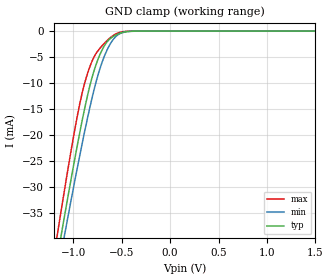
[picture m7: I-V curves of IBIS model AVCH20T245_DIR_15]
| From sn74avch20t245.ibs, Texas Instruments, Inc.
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[Model]   AVCH20T245_DIR_15
Model_type  Input
Vinl=0.49
Vinh=1.04
| variable   typ   min   max
C_comp   2.77pF   2.32pF   3.25pF
[Temperature Range]   40   100   -40
| Ambient temperature   25   85   -40
[Voltage range]   1.5   1.4   1.6
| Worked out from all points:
|   GND clamp passes 1 mA (typ) near -0.58 V on its own axis
[GND Clamp]
| AVCH20T245_DIR_15
|   Voltage   I(typ)   I(min)   I(max)
-4.6V     -459.2mA   -437.9mA   -484.2mA
-1.175V   -44.87mA   -48.03mA   -40.53mA
-1.145V   -41.6mA    -44.95mA   -37mA
-1.12V    -38.89mA   -42.4mA    -34.09mA
-1.095V   -36.21mA   -39.87mA   -31.21mA
-1.07V    -33.55mA   -37.35mA   -28.36mA
-945mV    -20.79mA   -25.16mA   -15.18mA
-840mV    -11.44mA   -15.71mA   -7.485mA
-775mV    -7.058mA   -10.58mA   -4.657mA
-700mV    -3.56mA    -5.9mA     -2.784mA
-545mV    -612.9uA   -811.6uA   -423.5uA
1.5V      118pA      793.8pA    21.88pA
